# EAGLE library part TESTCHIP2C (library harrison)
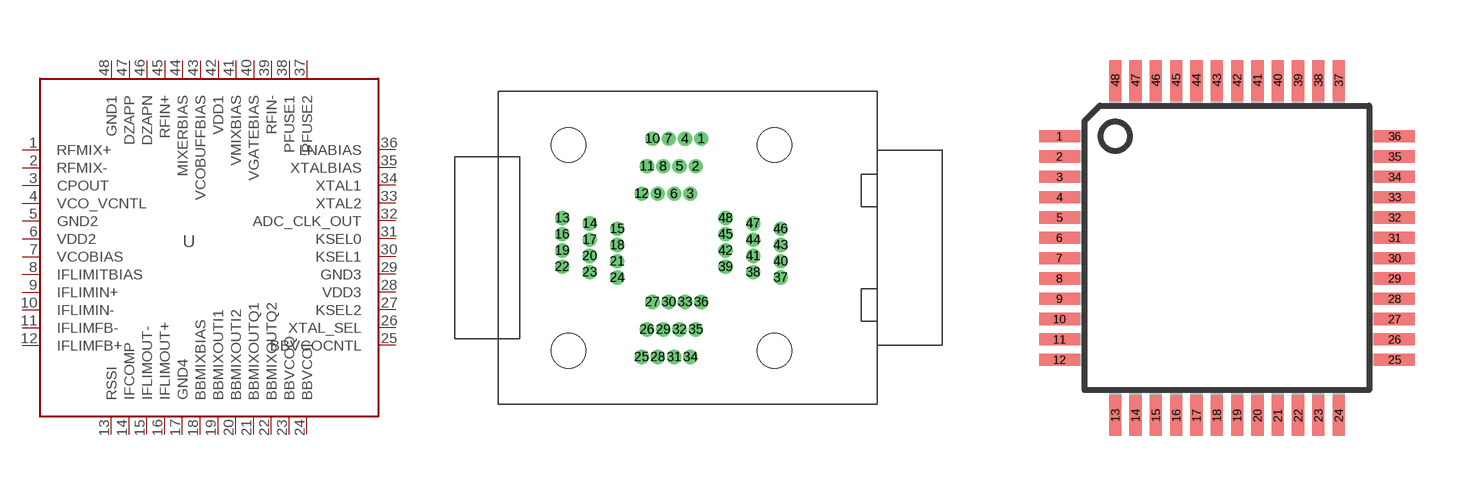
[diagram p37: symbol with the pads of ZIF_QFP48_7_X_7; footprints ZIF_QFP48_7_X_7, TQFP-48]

Designator prefix U

## TESTCHIP2CZIF  [ZIF_QFP48_7_X_7]
1  RFMIX+
2  RFMIX-
3  CPOUT
4  VCO_VCNTL
5  GND2
6  VDD2
7  VCOBIAS
8  IFLIMITBIAS
9  IFLIMIN+
10  IFLIMIN-
11  IFLIMFB-
12  IFLIMFB+
13  RSSI
14  IFCOMP
15  IFLIMOUT-
16  IFLIMOUT+
17  GND4
18  BBMIXBIAS
19  BBMIXOUTI1
20  BBMIXOUTI2
21  BBMIXOUTQ1
22  BBMIXOUTQ2
23  BBVCOQ
24  BBVCOI
25  BBVCOCNTL
26  XTAL_SEL
27  KSEL2
28  VDD3
29  GND3
30  KSEL1
31  KSEL0
32  ADC_CLK_OUT
33  XTAL2
34  XTAL1
35  XTALBIAS
36  LNABIAS
37  PFUSE2
38  PFUSE1
39  RFIN-
40  VGATEBIAS
41  VMIXBIAS
42  VDD1
43  VCOBUFFBIAS
44  MIXERBIAS
45  RFIN+
46  DZAPN
47  DZAPP
48  GND1

## TESTCHIP2CQFP  [TQFP-48]
Pads as for ZIF_QFP48_7_X_7

## Footprint ZIF_QFP48_7_X_7 (pad centres in mm)
drill 0.8 pad 1.27: 1 2.75,10.08; 2 2.25,7.54; 3 1.75,5; 4 1.25,10.08; 5 0.75,7.54; 6 0.25,5; 7 -0.25,10.08; 8 -0.75,7.54; 9 -1.25,5; 10 -1.75,10.08; 11 -2.25,7.54; 12 -2.75,5; 13 -10.08,2.75; 14 -7.54,2.25; 15 -5,1.75; 16 -10.08,1.25; 17 -7.54,0.75; 18 -5,0.25; 19 -10.08,-0.25; 20 -7.54,-0.75; 21 -5,-1.25; 22 -10.08,-1.75; 23 -7.54,-2.25; 24 -5,-2.75; 25 -2.75,-10.08; 26 -2.25,-7.54; 27 -1.75,-5; 28 -1.25,-10.08; 29 -0.75,-7.54; 30 -0.25,-5; 31 0.25,-10.08; 32 0.75,-7.54; 33 1.25,-5; 34 1.75,-10.08; 35 2.25,-7.54; 36 2.75,-5; 37 10.08,-2.75; 38 7.54,-2.25; 39 5,-1.75; 40 10.08,-1.25; 41 7.54,-0.75; 42 5,-0.25; 43 10.08,0.25; 44 7.54,0.75; 45 5,1.25; 46 10.08,1.75; 47 7.54,2.25; 48 5,2.75
hole 3.2 at 9.5,9.5
hole 3.2 at -9.5,9.5
hole 3.2 at -9.5,-9.5
hole 3.2 at 9.5,-9.5

## Footprint TQFP-48 (pad centres in mm)
smd 1.016 x 0.305: 1 -4.191,2.794; 2 -4.191,2.286; 3 -4.191,1.778; 4 -4.191,1.27; 5 -4.191,0.762; 6 -4.191,0.254; 7 -4.191,-0.254; 8 -4.191,-0.762; 9 -4.191,-1.27; 10 -4.191,-1.778; 11 -4.191,-2.286; 12 -4.191,-2.794; 25 4.191,-2.794; 26 4.191,-2.286; 27 4.191,-1.778; 28 4.191,-1.27; 29 4.191,-0.762; 30 4.191,-0.254; 31 4.191,0.254; 32 4.191,0.762; 33 4.191,1.27; 34 4.191,1.778; 35 4.191,2.286; 36 4.191,2.794
smd 0.305 x 1.016: 13 -2.794,-4.191; 14 -2.286,-4.191; 15 -1.778,-4.191; 16 -1.27,-4.191; 17 -0.762,-4.191; 18 -0.254,-4.191; 19 0.254,-4.191; 20 0.762,-4.191; 21 1.27,-4.191; 22 1.778,-4.191; 23 2.286,-4.191; 24 2.794,-4.191; 37 2.794,4.191; 38 2.286,4.191; 39 1.778,4.191; 40 1.27,4.191; 41 0.762,4.191; 42 0.254,4.191; 43 -0.254,4.191; 44 -0.762,4.191; 45 -1.27,4.191; 46 -1.778,4.191; 47 -2.286,4.191; 48 -2.794,4.191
